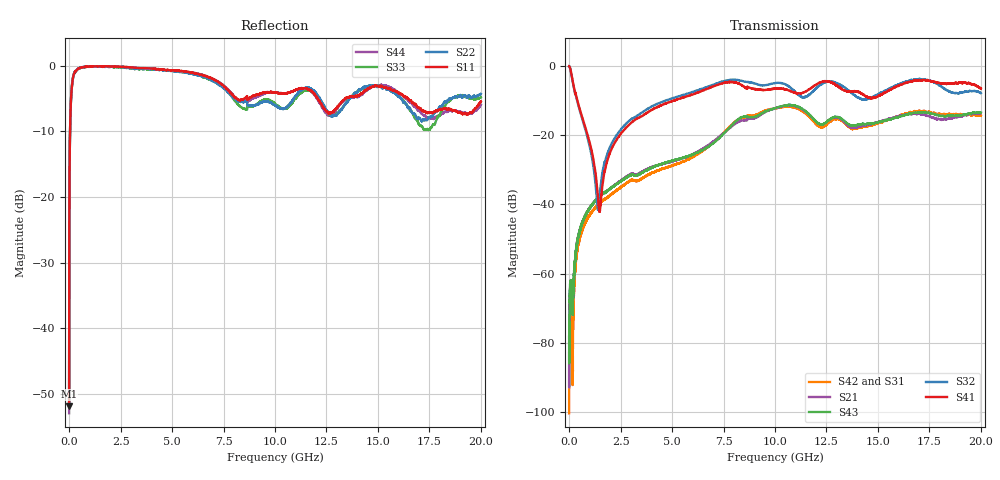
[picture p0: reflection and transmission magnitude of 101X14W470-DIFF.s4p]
! Created Wed Jul  6 17:22:56 2022
# khz S ma R 50
! 4 Port Network Data from SP2.SP block
! freq  magS11  angS11  magS12  angS12  magS13  angS13  magS14  angS14
!  magS21  angS21  magS22  angS22  magS23  angS23  magS24  angS24
!  magS31  angS31  magS32  angS32  magS33  angS33  magS34  angS34
!  magS41  angS41  magS42  angS42  magS43  angS43  magS44  angS44
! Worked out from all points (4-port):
!   20001 points, 300 kHz to 20 GHz, reference 50 ohm
!   strongest paths, dB at 300 kHz, 5 GHz, 10 GHz, 15 GHz, 20 GHz:
!     S41: 0.0, -10.1, -6.5, -8.7, -6.4
!     S32: -0.1, -9.3, -4.9, -8.2, -7.8
!     S43: -78.3, -27.4, -12.2, -16.3, -13.4
!     S21: -82.9, -27.5, -12.2, -16.2, -13.5
!     S42: -100.4, -28.8, -12.2, -16.6, -14.3
!     S31: -77.6, -28.7, -12.2, -16.6, -14.6
!   lowest |S11| = -51.9 dB at 300 kHz (marker M1), VSWR 1.01, Z = 49.9 - j0.244 ohm
!   |S11| at or under -10 dB: start of sweep to 45.6 MHz
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300  0.002554 -107.2  8.031e-05 -22.1  6.437e-05 83.2  0.9959 -0.1
     7.146e-05 73.0  0.002727 -102.0  0.9956 -0.1  0.0001225 169.0
     0.0001321 94.6  0.9916 -0.2  0.002582 -85.8  0.0001243 -174.7
     0.9995 -0.3  9.54e-06 65.6  0.0001221 -119.7  0.002252 -143.1
190300  0.8138 -146.3  0.0005143 99.0  0.0002179 105.5  0.5733 -55.8
        0.0005699 86.8  0.8172 -146.9  0.5665 -56.4  0.0001172 95.1
        0.0001657 141.9  0.5655 -56.3  0.8194 -147.0  0.0005472 102.9
        0.5743 -55.7  0.0001532 99.9  0.00044 95.4  0.8122 -146.3
541300  0.967 -171.1  0.004569 101.2  0.003567 104.6  0.2258 -79.5
        0.004484 102.4  0.9685 -172.1  0.2163 -80.0  0.003537 104.2
        0.003432 106.2  0.2168 -79.7  0.9622 -171.4  0.004466 100.8
        0.2257 -79.4  0.003505 104.3  0.004368 101.1  0.9681 -171.2
1483300  0.9935 169.8  0.01305 75.3  0.01035 75.2  0.007872 -7.7
         0.0131 75.0  0.9859 169.5  0.01342 41.8  0.01044 73.7
         0.01034 75.3  0.01361 41.7  0.9921 171.6  0.01316 75.7
         0.007851 -7.9  0.01035 73.9  0.01305 75.9  0.9905 169.4
2860300  0.9777 160.9  0.02607 58.9  0.02128 53.3  0.1377 65.1
         0.02614 58.5  0.9704 161.3  0.1565 64.1  0.0211 53.4
         0.02132 52.8  0.1568 64.4  0.9656 158.6  0.02532 56.3
         0.1374 65.0  0.02106 53.8  0.02529 56.3  0.9787 159.5
7404300  0.7253 115.4  0.1019 -32.9  0.1012 -43.9  0.5612 13.8
         0.1014 -32.8  0.6984 114.3  0.5927 10.1  0.1018 -40.8
         0.1013 -43.8  0.5943 10.2  0.7 107.3  0.09836 -38.9
         0.5611 13.8  0.102 -40.7  0.09793 -38.9  0.7299 114.1
2e7  0.5369 81.7  0.2106 9.1  0.1857 9.0  0.4727 -102.6
     0.211 8.8  0.612 75.2  0.4091 -91.6  0.1921 11.5
     0.1856 8.1  0.4085 -92.1  0.5745 68.7  0.2126 5.4
     0.4762 -103.5  0.1927 11.1  0.2137 5.5  0.5057 79.9
